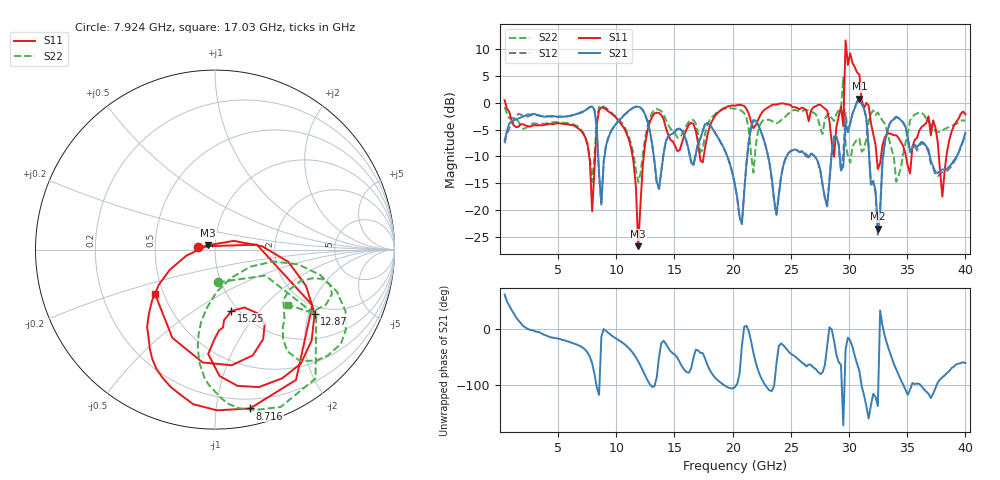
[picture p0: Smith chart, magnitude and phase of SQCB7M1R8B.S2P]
! Network Analyzer HP8722ES.07.66: Jul 25, 2000 Serial No. US39175408
! 26 Oct 2004  11:07:33
! Frequency  S11  S21  S12  S22
# HZ  S  DB R  50
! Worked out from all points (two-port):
!   201 points, 400 MHz to 40 GHz, reference 50 ohm
!   highest |S21| = 0.75 dB at 30.89 GHz (marker M1); lowest = -23.5 dB at 32.48 GHz (marker M2)
!   |S21| within 3 dB of the highest: 6.333 GHz to 8.181 GHz (1.848 GHz wide, 25.5 % of centre); 10.69 GHz to 12.49 GHz (1.798 GHz wide, 15.5 % of centre)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
!   lowest |S11| = -26.8 dB at 11.88 GHz (marker M3), VSWR 1.10, Z = 46.2 + j2.28 ohm
!   |S11| at or under -10 dB: 7.668 GHz to 8.182 GHz (514.7 MHz wide, 6.5 % of centre); 11.39 GHz to 12.36 GHz (965.4 MHz wide, 8.13 % of centre); 37.72 GHz to 38.37 GHz (647.2 MHz wide, 1.7 % of centre)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
!   |S22| runs from -14.8 to 4.7 dB; largest |S21 - S12| = 0.26
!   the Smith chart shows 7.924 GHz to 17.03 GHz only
!   S11 on the Smith chart (normalised r, x): 7.924 GHz: 0.82, +0.03; 8.716 GHz: 0.12, -1.24; 12.87 GHz: 1.74, -2.19; 15.25 GHz: 0.93, -0.73; 17.03 GHz: 0.45, -0.27
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4e8  0.48 -29.8  -7.03 61.3  -7.55 66.6  -0.77 -22.1
7.132e9  -5.70 -136.2  -1.63 -33.4  -1.71 -34.2  -5.51 -110.1
7.924e9  -20.25 169.9  -0.68 -61.3  -0.67 -61.6  -14.74 -85.1
8.716e9  -0.85 -77.6  -19.00 -13.8  -18.63 -11.8  -0.44 -67.4
1.1884e10  -26.75 147.6  -0.71 -57.9  -0.69 -58.1  -14.83 -60.4
1.2874e10  -3.61 -32.7  -5.16 -98.3  -5.26 -99.0  -2.88 -19.0
1.3666e10  -1.89 -72.3  -16.09 -50.7  -16.02 -48.6  -1.29 -43.4
1.525e10  -9.02 -75.1  -4.89 -51.5  -4.86 -51.7  -6.49 -36.4
1.7032e10  -7.62 -143.4  -7.52 -38.4  -7.43 -38.0  -5.84 -37.1
2.02e10  -0.54 -30.0  -15.39 -103.6  -15.30 -103.2  -1.11 -23.8
2.4358e10  -0.11 -40.8  -11.61 -29.0  -11.57 -29.0  -2.84 -178.9
2.6932e10  -0.83 -48.0  -9.74 -68.7  -9.73 -66.9  -1.82 88.1
2.9506e10  -4.34 12.5  -11.89 -172.0  -9.36 -144.5  4.71 18.5
2.9704e10  11.64 -28.9  -3.89 -36.2  -1.90 -19.6  -7.65 -36.0
3.01e10  9.24 -66.9  -3.87 -20.6  -3.73 -20.9  -11.19 43.7
3.0496e10  6.64 -84.4  -0.96 -48.3  -0.93 -47.7  -7.42 12.9
3.0694e10  5.66 75.4  0.30 -62.3  0.19 -61.6  -6.80 -178.9
3.0892e10  5.26 69.3  0.75 -75.6  0.55 -75.3  -6.67 168.4
3.1486e10  -0.01 -144.0  -2.83 -136.9  -2.84 -139.3  -6.67 -36.0
3.2476e10  -12.38 105.3  -23.49 -137.4  -24.63 -144.1  -1.79 -172.2
3.3466e10  -5.67 -25.7  -4.03 -39.2  -4.06 -40.3  -7.05 131.6
4e10  -2.15 65.4  -5.57 -60.8  -5.70 -59.6  -3.36 161.9
